|   This file is an IBIS representation of the   |
|   Texas Instruments   |
|   CDCVF857   |
|   48-DGG(TSSOP), 40-RTB(MLF) & 56-GQL(BGA) Packages   |
[IBIS Ver]   3.2
[File name]   cvf857_2.ibs
[File Rev]   0.2
[Date]   21 August 2003
[Source]   file originated at Texas Instruments
[Notes]   The following information corresponds to the
|   CDCVF857 output buffers and input ESD structures.
| Revision log:
| 01: 08/28/2003, initial version with updated driver model from CDCV857
|   To have a consisten temp range receiver plots were update
|   on temp information, but data was not changed.
| 02: 09/08/2003, Changed device name refrences from CDCVF857B to CDCVF857
|   kept internal names to have the reference to CDCVF857B-DIE
| NOTES:
| WARNINGS generated by Innoveda Visual IBIS Editor on Rising and Falling
| Waveforms are a best compromise for ramp resulution and TPD representation
| within the 100 data point limit.
| If rise/fall time analysis is more important then TPD, use the PLL-TYPE
| model which has better timing resolution. This is the default setting for
| this IBIS file.
| Some IBIS simulator(s) may need to be configured that options like
| "Strip V-t non switching time" is NOT checked (switched off) to get
| reasonable results on differential signal cross point.
| The start delay in the PLL-Type Model does not represent the phase between
| CLOCK and Yx. It has been set to its minimum value to plot the transitions.
| However, the shift in TPD between TYP/WEAK/STRONG has been minimized as it
| perfroms on a locked PLL.
[Disclaimer]
(C) Copyright Texas Instruments Incorporated 2003
   All rights reserved
  Texas Instruments Incorporated hereby grants the user of this IBIS
model a non-exclusive, nontransferable license to use this IBIS model
under the following terms.  Before using this IBIS model, the user
should read this license.  If the user does not accept these terms,
the IBIS model should be returned to Texas Instruments within 30 days.
  The user is granted this license only to use the IBIS model and
is not granted rights to sell, load, rent, lease or license the IBIS
model in whole or in part, or in modified form to anyone other than
user.  User may modify the IBIS model to suit its specific applications
but rights to derivative works and such modifications shall belong to
Texas Instruments.
  This IBIS model is provided on an "AS IS" basis and Texas Instruments
makes absolutely no warranty with respect to the information contained
herein.  TEXAS INSTRUMENTS DISCLAIMS AND CUSTOMER WAIVES ALL WARRANTIES,
EXPRESS OR IMPLIED, INCLUDING WARRANTIES OF MERCHANTABILITY OR FITNESS
FOR A PARTICULAR PURPOSE. The entire risk as to quality and performance
is with the Customer. ACCORDINGLY, IN NO EVENT SHALL THE COMPANY BE LIABLE
FOR ANY DAMAGES, WHETHER IN CONTRACT OR TORT,INCLUDING ANY LOST PROFITS
OR OTHER INCIDENTAL, CONSEQUENTIAL, EXEMPLARY, OR PUNITIVE DAMAGES ARISING
OUT OF THE USE OR APPLICATION OF THE IBIS model provided in this package.
Further, Texas Instruments reserves the right to discontinue or make changes
without notice to any product herein to improve reliability, function, or
design. Texas Instruments does not convey any license under patent rights
or any other intellectual property rights, including those of third parties.
Contact Texas Instruments at ATTN: HPA Department,
Texas Instruments 12500 TI blvd, M/S 8730, Dallas, TX 75243
IBIS Open Forum disclaims all warranties. See DISCLAIM.TXT
in vhdl.org:/pub/IBIS/models for the full disclaimer.
[Copyright]   Copyright 2003, Texas Instruments, All Rights Reserved
|=================== Component Section DGG -----------------------------------|
| Component CDCVF857DGG, 48-pin TSSOP
[Component]   CDCVF857DGG
[Manufacturer]  Texas Instruments Incorporated
[Package]
|   typ   min   max
R_pkg   0.225hm   0.199Ohm   0.255Ohm
L_pkg   4.851nH   4.027nH   5.945nH
C_pkg   0.336pF   0.204pF   0.751pF
[Pin] signal_name   model_name   R_Pin   L_Pin   C_Pin
  1   GND   GND   0.222Ohm   5.869nH   0.751pF
  2   Y0-   CDCVF857B_DOUT   0.226Ohm   5.621nH   0.493pF
  3   Y0   CDCVF857B_DOUT   0.232Ohm   5.425nH   0.395pF
  4   VCC   POWER   0.236Ohm   5.171nH   0.371pF
  5   Y1   CDCVF857B_DOUT   0.252Ohm   5.208nH   0.348pF
  6   Y1-   CDCVF857B_DOUT   0.249Ohm   5.041nH   0.345pF
  7   GND   GND   0.237Ohm   4.781nH   0.265pF
  8   GND   GND   0.225Ohm   4.607nH   0.256pF
  9   Y2-   CDCVF857B_DOUT   0.214Ohm   4.377nH   0.238pF
 10   Y2   CDCVF857B_DOUT   0.208Ohm   4.249nH   0.225pF
 11   VCC   POWER   0.203Ohm   4.118nH   0.217pF
 12   VCC   POWER   0.202Ohm   4.084nH   0.205pF
 13   CLK   CDCVF857B_CLKIN   0.203Ohm   4.090nH   0.208pF
 14   CLK-   CDCVF857B_CLKIN   0.204Ohm   4.121nH   0.216pF
 15   VCC   POWER   0.207Ohm   4.209nH   0.227pF
 16   AVCC   POWER   0.212Ohm   4.338nH   0.238pF
 17   AGND   GND   0.221Ohm   4.535nH   0.248pF
 18   GND   GND   0.235Ohm   4.764nH   0.304pF
 19   Y3-   CDCVF857B_DOUT   0.248Ohm   5.064nH   0.346pF
 20   Y3   CDCVF857B_DOUT   0.255Ohm   5.195nH   0.385pF
 21   VCC   POWER   0.240Ohm   5.211nH   0.393pF
 22   Y4   CDCVF857B_DOUT   0.231Ohm   5.397nH   0.468pF
 23   Y4-   CDCVF857B_DOUT   0.228Ohm   5.648nH   0.531pF
 24   GND   GND   0.223Ohm   5.913nH   0.413pF
 25   GND   GND   0.222Ohm   5.848nH   0.749pF
 26   Y9-   CDCVF857B_DOUT   0.223Ohm   5.542nH   0.490pF
 27   Y9   CDCVF857B_DOUT   0.228Ohm   5.318nH   0.393pF
 28   VCC   POWER   0.237Ohm   5.127nH   0.368pF
 29   Y8   CDCVF857B_DOUT   0.249Ohm   5.087nH   0.316pF
 30   Y8-   CDCVF857B_DOUT   0.248Ohm   5.018nH   0.335pF
 31   GND   GND   0.235Ohm   4.761nH   0.300pF
 32   FBOUT   CDCVF857B_DOUT   0.220Ohm   4.485nH   0.253pF
 33   FBOUT-   CDCVF857B_DOUT   0.210Ohm   4.299nH   0.235pF
 34   VCC   POWER   0.204Ohm   4.152nH   0.223pF
 35   FBIN-   CDCVF857B_CLKIN   0.200Ohm   4.050nH   0.214pF
 36   FBIN   CDCVF857B_CLKIN   0.199Ohm   4.027nH   0.204pF
 37   PWRDWN   CDCVF857B_PWRDWN   0.200Ohm   4.030nH   0.208pF
 38   VCC   POWER   0.200Ohm   4.041nH   0.211pF
 39   Y7   CDCVF857B_DOUT   0.203Ohm   4.160nH   0.227pF
 40   Y7-   CDCVF857B_DOUT   0.210Ohm   4.308nH   0.240pF
 41   GND   GND   0.220Ohm   4.486nH   0.245pF
 42   GND   GND   0.235Ohm   4.758nH   0.306pF
 43   Y6-   CDCVF857B_DOUT   0.247Ohm   5.034nH   0.343pF
 44   Y6   CDCVF857B_DOUT   0.252Ohm   5.129nH   0.381pF
 45   VCC   POWER   0.241Ohm   5.207nH   0.395pF
 46   Y5   CDCVF857B_DOUT   0.230Ohm   5.366nH   0.470pF
 47   Y5-   CDCVF857B_DOUT   0.227Ohm   5.625nH   0.533pF
 48   GND   GND   0.224Ohm   5.945nH   0.410pF
[Diff_Pin]  inv_pin  vdiff   tdelay_typ  tdelay_min  tdelay_max
| The '+' pin is   Diff_pin,   the '-' pin is the   Inv_pin
| Receiver Pins  |  Receiver Vth = +/-200mV
13   14   0.2   0ns   0ns   0ns   | CLK  / CLK-
36   35   0.2   0ns   0ns   0ns   | FBIN / FBIN-
| Driver Pins   |  Rload = 60 OHM to VCC/2 termination
32   33   NA   0ns   0ns   0ns   | FBOUT / FBOUT-
3   2   NA   0ns   0ns   0ns   | Y0 / Y0-
5   6   NA   0ns   0ns   0ns   | Y1 / Y1-
10   9   NA   0ns   0ns   0ns   | Y2 / Y2-
20   19   NA   0ns   0ns   0ns   | Y3 / Y3-
22   23   NA   0ns   0ns   0ns   | Y4 / Y4-
46   47   NA   0ns   0ns   0ns   | Y5 / Y5-
44   43   NA   0ns   0ns   0ns   | Y6 / Y6-
39   40   NA   0ns   0ns   0ns   | Y7 / Y7-
29   30   NA   0ns   0ns   0ns   | Y8 / Y8-
27   26   NA   0ns   0ns   0ns   | Y9 / Y9-
[Model Selector]   CDCVF857B_DOUT
CDCVF857B_PLL for PLL_MODE (no buffer delay, no shift between TYP,MIN,MAX in VT)
CDCVF857B_BUF for SIMPLE_BUFFER_MODE (real buffer delay in VT table)
|================== Component Section MLF ------------------------------------|
| Component CDCVF857RTB, 40-pin MLF
[Component]   CDCVF857RTB
[Manufacturer]  Texas Instruments
[Package]
|   typ   min   max
R_pkg   0.125Ohm   0.069Ohm   0.161Ohm
L_pkg   1.178nH   0.596nH   1.594nH
C_pkg   0.067pF   0.025pF   0.159pF
[Pin] signal_name  model_name   R_Pin   L_Pin   C_Pin
  1   GND   GND   0.151Ohm   1.478nH   0.095pF
  2   Y2-   CDCVF857B_DOUT1   0.148Ohm   1.432nH   0.080pF
  3   Y2   CDCVF857B_DOUT1   0.141Ohm   1.356nH   0.111pF
  4   VDDQ   POWER   0.069Ohm   0.657nH   0.159pF
  5   CLK   CDCVF857B_CLKIN   0.135Ohm   1.285nH   0.070pF
  6   CLK-   CDCVF857B_CLKIN   0.134Ohm   1.270nH   0.071pF
  7   VDDQ   POWER   0.135Ohm   1.286nH   0.072pF
  8   AVVD   POWER   0.139Ohm   1.331nH   0.074pF
  9   AGND   GND   0.145Ohm   1.400nH   0.078pF
 10   GND   GND   0.152Ohm   1.488nH   0.071pF
 11   Y3-   CDCVF857B_DOUT1   0.145Ohm   1.413nH   0.048pF
 12   Y3   CDCVF857B_DOUT1   0.125Ohm   1.186nH   0.085pF
 13   VDDQ   POWER   0.115Ohm   1.067nH   0.063pF
 14   Y4   CDCVF857B_DOUT1   0.111Ohm   1.019nH   0.056pF
 15   Y4-   CDCVF857B_DOUT1   0.109Ohm   1.005nH   0.055pF
 16   Y9-   CDCVF857B_DOUT1   0.109Ohm   1.002nH   0.056pF
 17   Y9   CDCVF857B_DOUT1   0.111Ohm   1.019nH   0.057pF
 18   VDDQ   POWER   0.115Ohm   1.073nH   0.054pF
 19   Y8   CDCVF857B_DOUT1   0.126Ohm   1.192nH   0.076pF
 20   Y8-   CDCVF857B_DOUT1   0.145Ohm   1.418nH   0.077pF
 21   FBOUT   CDCVF857B_DOUT1   0.156Ohm   1.539nH   0.084pF
 22   FBOUT-   CDCVF857B_DOUT1   0.148Ohm   1.438nH   0.073pF
 23   VDDQ   POWER   0.141Ohm   1.360nH   0.061pF
 25   FBIN-   CDCVF857B_CLKIN   0.134Ohm   1.274nH   0.073pF
 26   FBIN   CDCVF857B_CLKIN   0.136Ohm   1.289nH   0.070pF
 27   PWRDWN-  CDCVF857B_PWRDWN   0.139Ohm   1.332nH   0.074pF
 28   VDDQ   POWER   0.145Ohm   1.401nH   0.075pF
 29   Y7   CDCVF857B_DOUT1   0.152Ohm   1.489nH   0.081pF
 30   Y7-   CDCVF857B_DOUT1   0.161Ohm   1.594nH   0.041pF
 31   Y6-   CDCVF857B_DOUT1   0.145Ohm   1.405nH   0.081pF
 32   Y6   CDCVF857B_DOUT1   0.125Ohm   1.178nH   0.097pF
 33   VDDQ   POWER   0.115Ohm   1.059nH   0.060pF
 34   Y5   CDCVF857B_DOUT1   0.110Ohm   1.010nH   0.049pF
 35   Y5-   CDCVF857B_DOUT1   0.109Ohm   0.996nH   0.054pF
 36   Y0-   CDCVF857B_DOUT1   0.109Ohm   0.994nH   0.049pF
 37   Y0   CDCVF857B_DOUT1   0.111Ohm   1.011nH   0.033pF
 38   VDDQ   POWER   0.115Ohm   1.064nH   0.025pF
 39   Y1   CDCVF857B_DOUT1   0.126Ohm   1.184nH   0.101pF
 40   Y1-   CDCVF857B_DOUT1   0.145Ohm   1.409nH   0.084pF
PAD   GND   GND   0.011Ohm   0.093nH   0.316pF
[Diff_Pin]  inv_pin  vdiff   tdelay_typ  tdelay_min  tdelay_max
| The '+' pin is   Diff_pin,   the '-' pin is the   Inv_pin
| Receiver Pins  |  Receiver Vth = +/-200mV
 5   6   0.2   0ns   0ns   0ns   | CLK  / CLK-
26   25   0.2   0ns   0ns   0ns   | FBIN / FBIN-
| Driver Pins   |  Rload = 60 OHM to VCC/2 termination
 3   2   NA   0ns   0ns   0ns   | Y2 / Y2-
12   11   NA   0ns   0ns   0ns   | Y3 / Y3-
14   15   NA   0ns   0ns   0ns   | Y4 / Y4-
17   16   NA   0ns   0ns   0ns   | Y9 / Y9-
19   20   NA   0ns   0ns   0ns   | Y8 / Y8-
21   22   NA   0ns   0ns   0ns   | FBOUT / FBOUT-
29   30   NA   0ns   0ns   0ns   | Y7 / Y7-
32   31   NA   0ns   0ns   0ns   | Y6 / Y6-
34   35   NA   0ns   0ns   0ns   | Y5 / Y5-
37   36   NA   0ns   0ns   0ns   | Y0 / Y0-
39   40   NA   0ns   0ns   0ns   | Y1 / Y1-
[Model Selector]   CDCVF857B_DOUT1
CDCVF857B_PLL for PLL_MODE (no buffer delay, no shift between TYP,MIN,MAX in VT)
CDCVF857B_BUF for SIMPLE_BUFFER_MODE (real buffer delay in VT table)
|=================== Component Section GQL -----------------------------------|
| Component CDCVF857GQL, 56-pin GQL
[Component]   CDCVF857GQL
[Manufacturer]  Texas Instruments Incorporated
[Package]
|   typ   min   max
R_pkg   0.243hm   0.191Ohm   0.327Ohm
L_pkg   3.781nH   3.014nH   5.677nH
C_pkg   0.207pF   0.100pF   0.370pF
[Pin] signal_name  model_name   R_Pin   L_Pin   C_Pin
 A3   GND   GND   0.251Ohm   3.326nH   0.159pF
 A2   Y0-   CDCVF857B_DOUT2   0.260Ohm   3.575nH   0.163pF
 A1   Y0   CDCVF857B_DOUT2   0.279Ohm   3.914nH   0.174pF
 B3   VCC   POWER   0.327Ohm   5.677nH   0.370pF
 B2   Y1   CDCVF857B_DOUT2   0.278Ohm   4.430nH   0.242pF
 B1   Y1-   CDCVF857B_DOUT2   0.253Ohm   3.802nH   0.099pF
|C3   NC   0.085Ohm   2.691nH   0.181pF
 C2   GND   GND   0.247Ohm   4.027nH   0.279pF
 C1   GND   GND   0.226Ohm   3.461nH   0.204pF
 D2   Y2-   CDCVF857B_DOUT2   0.234Ohm   3.846nH   0.166pF
|D3   NC   0.091Ohm   2.924nH   0.224pF
 D1   Y2   CDCVF857B_DOUT2   0.204Ohm   3.175nH   0.272pF
 E2   VCC   POWER   0.206Ohm   3.516nH   0.158pF
 E1   VCC   POWER   0.193Ohm   3.018nH   0.202pF
 F1   CLK   CDCVF857B_CLKIN   0.193Ohm   3.014nH   0.134pF
 F2   CLK-   CDCVF857B_CLKIN   0.206Ohm   3.502nH   0.175pF
 G1   VCC   POWER   0.203Ohm   3.150nH   0.210pF
|G3   NC   0.092Ohm   2.917nH   0.162pF
 G2   AVCC   POWER   0.235Ohm   3.838nH   0.324pF
 H1   AGND   GND   0.226Ohm   3.427nH   0.197pF
 H2   GND   GND   0.243Ohm   3.942nH   0.162pF
|H3   NC   0.086Ohm   2.664nH   0.219pF
 J1   Y3-   CDCVF857B_DOUT2   0.191Ohm   3.105nH   0.255pF
 J2   Y3   CDCVF857B_DOUT2   0.271Ohm   4.370nH   0.158pF
 J3   VCC   POWER   0.316Ohm   5.605nH   0.238pF
 K1   Y4   CDCVF857B_DOUT2   0.269Ohm   3.806nH   0.340pF
 K2   Y4-   CDCVF857B_DOUT2   0.255Ohm   3.561nH   0.149pF
 K3   GND   GND   0.249Ohm   3.330nH   0.131pF
 K4   GND   GND   0.249Ohm   3.323nH   0.121pF
 K5   Y9-   CDCVF857B_DOUT2   0.255Ohm   3.538nH   0.142pF
 K6   Y9   CDCVF857B_DOUT2   0.273Ohm   3.855nH   0.156pF
 J4   VCC   POWER   0.318Ohm   5.624nH   0.171pF
 J5   Y8   CDCVF857B_DOUT2   0.279Ohm   4.436nH   0.364pF
 J6   Y8-   CDCVF857B_DOUT2   0.253Ohm   3.774nH   0.252pF
|H4   NC   0.085Ohm   2.658nH   0.179pF
 H5   GND   GND   0.248Ohm   4.017nH   0.279pF
 H6   FBOUT   CDCVF857B_DOUT2   0.226Ohm   3.423nH   0.206pF
 G5   FBOUT-   CDCVF857B_DOUT2   0.235Ohm   3.838nH   0.165pF
|G4   NC   0.092Ohm   2.922nH   0.223pF
 G6   VCC   POWER   0.204Ohm   3.150nH   0.272pF
 F5   FBIN-   CDCVF857B_CLKIN   0.206Ohm   3.502nH   0.158pF
 F6   FBIN   CDCVF857B_CLKIN   0.193Ohm   3.016nH   0.203pF
 E6   PWRDWN   CDCVF857B_PWRDWN   0.193Ohm   3.018nH   0.132pF
 E5   VCC   POWER   0.206Ohm   3.511nH   0.178pF
 D6   Y7   CDCVF857B_DOUT2   0.204Ohm   3.166nH   0.213pF
|D4   NC   0.092Ohm   2.933nH   0.164pF
 D5   Y7-   CDCVF857B_DOUT2   0.234Ohm   3.851nH   0.321pF
 C6   GND   GND   0.225Ohm   3.436nH   0.195pF
 C5   GND   GND   0.245Ohm   4.036nH   0.164pF
|C4   NC   0.086Ohm   2.675nH   0.230pF
 B6   Y6-   CDCVF857B_DOUT2   0.253Ohm   3.778nH   0.249pF
 B5   Y6   CDCVF857B_DOUT2   0.279Ohm   4.492nH   0.159pF
 B4   VCC   POWER   0.324Ohm   5.655nH   0.242pF
 A6   Y5   CDCVF857B_DOUT2   0.253Ohm   3.668nH   0.340pF
 A5   Y5-   CDCVF857B_DOUT2   0.260Ohm   3.600nH   0.158pF
 A4   GND   GND   0.251Ohm   3.351nH   0.135pF
[Diff_Pin]  inv_pin  vdiff   tdelay_typ  tdelay_min  tdelay_max
| The '+' pin is   Diff_pin,   the '-' pin is the   Inv_pin
| Receiver Pins  |  Receiver Vth = +/-200mV
F1   F2   0.2   0ns   0ns   0ns   | CLK  / CLK-
F6   F5   0.2   0ns   0ns   0ns   | FBIN / FBIN-
| Driver Pins   |  Rload = 60 OHM to VCC/2 termination
H6   G5   NA   0ns   0ns   0ns   | FBOUT / FBOUT-
A1   A2   NA   0ns   0ns   0ns   | Y0 / Y0-
B2   B1   NA   0ns   0ns   0ns   | Y1 / Y1-
D1   D2   NA   0ns   0ns   0ns   | Y2 / Y2-
J2   J1   NA   0ns   0ns   0ns   | Y3 / Y3-
K1   K2   NA   0ns   0ns   0ns   | Y4 / Y4-
A6   A5   NA   0ns   0ns   0ns   | Y5 / Y5-
B5   B6   NA   0ns   0ns   0ns   | Y6 / Y6-
D6   D5   NA   0ns   0ns   0ns   | Y7 / Y7-
J5   J6   NA   0ns   0ns   0ns   | Y8 / Y8-
K6   K5   NA   0ns   0ns   0ns   | Y9 / Y9-
[Model Selector]  CDCVF857B_DOUT2
CDCVF857B_PLL for PLL_MODE (no buffer delay, no shift between TYP,MIN,MAX in VT)
CDCVF857B_BUF for SIMPLE_BUFFER_MODE (real buffer delay in VT table)
|--------------------- End of Component Section--------------------------------|
| Models and submodels in the file (4): CDCVF857B_PWRDWN (Input), CDCVF857B_CLKIN (Input), CDCVF857B_PLL (3-state), CDCVF857B_BUF (3-state)
